[IBIS VER]   5.0
[File Name]   am13e230pzh.ibs
[File Rev]   1.0
[Date]   February 08, 2026
[Source]   File originated at Texas Instruments
[Copyright]   (c) 2012, Texas Instruments Inc.
[Component]   am13e230pzh
[Manufacturer] Texas Instruments
[Package]
| Variable   Typ   Min   Max
   R_pkg 3.31E-01 5.89E-02 4.13E-01
   L_pkg 7.43E-09 3.45E-09 1.00E-08
   C_pkg 1.76E-14 8.71E-15 4.53E-14
[Pin]   signal_name   model_name   R_pin   L_pin   C_pin
   1   PC2   BCF3385DSHYPBFZSD_87U 3.83E-01 8.46E-09 3.97E-14
   2   PC3   BCF3385DSHYPBFZSD_87U 3.62E-01 8.13E-09 1.93E-14
   3   PC4   BCF3385DSHYPBFZSD_87U 3.50E-01 7.91E-09 1.88E-14
   4   PC5   BCF3385DSHYPBFZSD_87U 3.41E-01 7.70E-09 1.83E-14
   5   PC6   BCF3385DSWHYPBFZSD_87U 3.34E-01 7.52E-09 1.78E-14
   6   VDD   NC 3.34E-01 7.42E-09 1.74E-14
   7   PB13   BCF3385DSWHYPBFZSD_87U 3.26E-01 7.22E-09 1.70E-14
   8   PB14   BCF3385DSHYPBFZSD_87U 3.24E-01 7.10E-09 1.66E-14
   9   PB15   BCF3385DSHYPBFZSD_87U 3.23E-01 6.98E-09 1.61E-14
   10   VSS   NC 3.28E-01 6.93E-09 1.58E-14
   11   VDD   NC 3.30E-01 6.83E-09 1.54E-14
   12 PC16_X1   BCF3385DSHYPBFZSD_87U 3.24E-01 6.67E-09 1.81E-14
   13 PC17_X2   BCF3385DSHYPBFZSD_87U 3.22E-01 6.54E-09 1.76E-14
   14   NRST   BQ0491FSSD_XRSN_87U 3.25E-01 6.67E-09 1.81E-14
   15   PB0   BCF3385DSHYPBFZSD_87U 3.27E-01 6.80E-09 1.54E-14
   16   PB1   BCF3385DSWHYPBFZSD_87U 3.30E-01 6.94E-09 1.58E-14
   17   PB2   BCF3385DSHYPBFZSD_87U 3.34E-01 7.09E-09 1.62E-14
   18   PB3   BCF3385DSHYPBFZSD_87U 3.40E-01 7.26E-09 1.67E-14
   19   VSS   NC 3.52E-01 7.50E-09 1.72E-14
   20   VREFLO   NC 3.59E-01 7.67E-09 1.76E-14
   21   VREFHI   NC 3.56E-01 7.75E-09 1.80E-14
   22   VREFHI   NC 3.67E-01 7.97E-09 1.85E-14
   23   PA0   BCF3385DSWHYPBFZSD_87U 3.76E-01 8.17E-09 1.90E-14
   24   PA1   BCF3385DSHYPBFZSD_87U 3.89E-01 8.41E-09 1.95E-14
   25   PA2   BCF3385DSWHYPBFZSD_87U 4.05E-01 8.68E-09 4.00E-14
   26   PA3   BCF3385DSHYPBFZSD_87U 3.95E-01 1.00E-08 2.20E-14
   27   VSSA   NC 2.08E-01 7.97E-09 1.32E-14
   28   VDDA   NC 2.02E-01 7.77E-09 1.29E-14
   29   PA4   BCF3385DSHYPBFZSD_87U 3.48E-01 9.13E-09 1.01E-14
   30   PA5   BCF3385DSHYPBFZSD_87U 3.39E-01 8.90E-09 9.80E-15
   31   PA6   BCF3385DSHYPBFZSD_87U 3.33E-01 8.69E-09 9.56E-15
   32   PA7   BCF3385DSHYPBFZSD_87U 3.27E-01 8.49E-09 9.33E-15
   33   PB4   BCF3385DSHYPBFZSD_87U 3.24E-01 8.31E-09 9.11E-15
   34   PB5   BCF3385DSWHYPBFZSD_87U 3.22E-01 8.15E-09 8.90E-15
   35   PA16   BCF3385DSHYPBFZSD_87U 3.21E-01 8.00E-09 8.71E-15
   36   PA17   BCF3385DSHYPBFZSD_87U 3.22E-01 7.86E-09 1.95E-14
   37   PA18   BCF3385DSHYPBFZSD_87U 3.24E-01 7.74E-09 1.90E-14
   38   PC7   BCF3385DSHYPBFZSD_87U 3.27E-01 7.63E-09 1.85E-14
   39   PC8   BCF3385DSHYPBFZSD_87U 3.22E-01 7.44E-09 1.79E-14
   40   PC9   BCF3385DSHYPBFZSD_87U 3.18E-01 7.25E-09 1.73E-14
   41   PC10   BCF3385DSHYPBFZSD_87U 3.15E-01 7.08E-09 1.68E-14
   42   PC11   BCF3385DSHYPBFZSD_87U 3.14E-01 6.93E-09 1.62E-14
   43   PC12   BCF3385DSHYPBFZSD_87U 3.15E-01 6.80E-09 1.57E-14
   44   PC13   BCF3385DSHYPBFZSD_87U 3.17E-01 6.68E-09 1.52E-14
   45   PC14   BCF3385DSHYPBFZSD_87U 3.21E-01 6.58E-09 1.78E-14
   46   PC15   BCF3385DSHYPBFZSD_87U 3.27E-01 6.49E-09 1.72E-14
   47   PA26   BCF3385DSHYPBFZSD_87U 3.34E-01 6.43E-09 1.66E-14
   48   NC   NC 5.89E-02 3.45E-09 1.38E-14
   49   VSS   NC 1.91E-01 4.66E-09 1.81E-14
   50   VDD   NC 3.69E-01 6.72E-09 2.96E-14
   51   PA28   BCF3385DSHYPBFZSD_87U 3.84E-01 8.47E-09 3.97E-14
   52   PA29   BCF3385DSHYPBFZSD_87U 3.71E-01 8.22E-09 1.93E-14
   53   PA30   BCF3385DSHYPBFZSD_87U 3.59E-01 8.00E-09 1.88E-14
   54   PA31   BCF3385DSHYPBFZSD_87U 3.49E-01 7.79E-09 1.84E-14
   55   PB24   BCF3385DSHYPBFZSD_87U 3.44E-01 7.62E-09 1.79E-14
   56   PB25   BCF3385DSHYPBFZSD_87U 3.37E-01 7.45E-09 1.75E-14
   57   PB26   BCF3385DSHYPBFZSD_87U 3.32E-01 7.29E-09 1.70E-14
   58   PB27   BCF3385DSHYPBFZSD_87U 3.28E-01 7.14E-09 1.66E-14
   59   PB28   BCF3385DSHYPBFZSD_87U 3.26E-01 7.01E-09 1.62E-14
   60   PB29   BCF3385DSHYPBFZSD_87U 3.24E-01 6.89E-09 1.58E-14
   61   PB30   BCF3385DSHYPBFZSD_87U 3.23E-01 6.77E-09 1.53E-14
   62   PB31   BCF3385DSHYPBFZSD_87U 3.24E-01 6.67E-09 1.81E-14
   63   PB6   BCF3385DSHYPBFZSD_87U 3.25E-01 6.57E-09 1.76E-14
   64   PB7   BCF3385DSHYPBFZSD_87U 3.27E-01 6.70E-09 1.81E-14
   65   PB8   BCF3385DSHYPBFZSD_87U 3.25E-01 6.79E-09 1.54E-14
   66   PB9   BCF3385DSHYPBFZSD_87U 3.28E-01 6.92E-09 1.58E-14
   67   PA8   BCF3385DSHYPBFZSD_87U 3.32E-01 7.07E-09 1.62E-14
   68   PA9   BCF3385DSHYPBFZSD_87U 3.37E-01 7.24E-09 1.67E-14
   69   PA10   BCF3385DSHYPBFZSD_87U 3.44E-01 7.41E-09 1.71E-14
   70   PA11   BCF3385DSHYPBFZSD_87U 3.40E-01 7.48E-09 1.75E-14
   71   PA12  BCPF335585DSHYPBFZSD_87U 3.48E-01 7.67E-09 1.80E-14
   72   PA13 BCF3385DSHYPBFZSD_TMS_87U 3.49E-01 7.78E-09 1.84E-14
   73   PC22   BCF3385DSHYPBFZSD_87U 3.59E-01 7.99E-09 1.88E-14
   74   VSS   NC 3.76E-01 8.28E-09 1.94E-14
   75   VDD   NC 2.10E-01 6.68E-09 4.53E-14
   76   PA14 BCF3385DSHYPBFZSD_TMS_87U 3.87E-01 9.96E-09 2.18E-14
   77   PA15  BCPF335585DSHYPBFZSD_87U 3.72E-01 9.67E-09 1.06E-14
   78   PB10   BCF3385DSHYPBFZSD_87U 3.60E-01 9.39E-09 1.03E-14
   79   PB11   BCF3385DSHYPBFZSD_87U 3.49E-01 9.14E-09 1.01E-14
   80   PB12   BCF3385DSHYPBFZSD_87U 3.40E-01 8.91E-09 9.80E-15
   81   PB16   BCF3385DSHYPBFZSD_87U 3.44E-01 8.80E-09 9.64E-15
   82   PB17   BCF3385DSHYPBFZSD_87U 3.36E-01 8.58E-09 9.39E-15
   83   PB18  BCPF335585DSHYPBFZSD_87U 3.35E-01 8.43E-09 9.20E-15
   84   PB19   BCF3385DSWHYPBFZSD_87U 3.31E-01 8.25E-09 8.98E-15
   85   PB20   BCF3385DSHYPBFZSD_87U 3.27E-01 8.06E-09 8.75E-15
   86   PB21   BCF3385DSHYPBFZSD_87U 3.23E-01 7.88E-09 1.95E-14
   87   PB22   BCF3385DSHYPBFZSD_87U 3.21E-01 7.72E-09 1.90E-14
   88   PB23   BCF3385DSHYPBFZSD_87U 3.21E-01 7.57E-09 1.84E-14
   89   PA19  BCPF335585DSHYPBFZSD_87U 3.20E-01 7.42E-09 1.79E-14
   90   PA20   BCF3385DSHYPBFZSD_87U 3.21E-01 7.28E-09 1.74E-14
   91   PA21   BCF3385DSHYPBFZSD_87U 3.20E-01 7.13E-09 1.68E-14
   92   PA22   BCF3385DSHYPBFZSD_87U 3.22E-01 7.01E-09 1.63E-14
   93   PA23   BCF3385DSHYPBFZSD_87U 3.26E-01 6.91E-09 1.58E-14
   94   PD11   BCF3385DSHYPBFZSD_87U 3.31E-01 6.82E-09 1.53E-14
   95   PA24   BCF3385DSHYPBFZSD_87U 3.38E-01 6.75E-09 1.79E-14
   96   PA25   BCF3385DSHYPBFZSD_87U 3.46E-01 6.69E-09 1.73E-14
   97   PC0   BCF3385DSHYPBFZSD_87U 3.56E-01 6.65E-09 1.67E-14
   98   PC1   BCF3385DSHYPBFZSD_87U 3.68E-01 6.64E-09 1.62E-14
   99   VSS   NC 2.01E-01 4.77E-09 1.84E-14
   100   VDD   NC 4.01E-01 7.05E-09 3.01E-14
| End of package information
|   Component BCF3385DSHYPBFZSD_87U
[Component] BCF3385DSHYPBFZSD_87U
[Manufacturer] Texas Instruments
[Package]
| variable   typ   min   max
R_pkg   0.0   0.0   0.0
L_pkg   0.0H   0.0H   0.0H
C_pkg   0.0F   0.0F   0.0F
[Pin]  signal_name   model_name   R_pin   L_pin   C_pin
PAD   PAD   BCF3385DSHYPBFZSD_87U
VDDS   VDDS   Power
VSS   VSS   Gnd
A   A   NC
GZ   GZ   NC
[Model Selector] BCF3385DSHYPBFZSD_87U
BCF3385DSHYPBFZSD_87U_PUPDOFF PI=1 PSEL=1
BCF3385DSHYPBFZSD_87U_PDON PI=0 PSEL=0
BCF3385DSHYPBFZSD_87U_PUON PI=0 PSEL=1
|   Component BCF3385DSHYPBFZSD_TMS_87U
[Component] BCF3385DSHYPBFZSD_TMS_87U
[Manufacturer] Texas Instruments
[Package]
| variable   typ   min   max
R_pkg   0.0   0.0   0.0
L_pkg   0.0H   0.0H   0.0H
C_pkg   0.0F   0.0F   0.0F
[Pin]  signal_name   model_name   R_pin   L_pin   C_pin
PAD   PAD   BCF3385DSHYPBFZSD_TMS_87U
VDDS   VDDS   Power
VSS   VSS   Gnd
A   A   NC
GZ   GZ   NC
[Model Selector] BCF3385DSHYPBFZSD_TMS_87U
BCF3385DSHYPBFZSD_TMS_87U_PUPDOFF PI=1 PSEL=1
BCF3385DSHYPBFZSD_TMS_87U_PDON PI=0 PSEL=0
BCF3385DSHYPBFZSD_TMS_87U_PUON PI=0 PSEL=1
|   Component BCF3385DSWHYPBFZSD_87U
[Component] BCF3385DSWHYPBFZSD_87U
[Manufacturer] Texas Instruments
[Package]
| variable   typ   min   max
R_pkg   0.0   0.0   0.0
L_pkg   0.0H   0.0H   0.0H
C_pkg   0.0F   0.0F   0.0F
[Pin]  signal_name   model_name   R_pin   L_pin   C_pin
PAD   PAD   BCF3385DSWHYPBFZSD_87U
VDDS   VDDS   Power
VSS   VSS   Gnd
A   A   NC
GZ   GZ   NC
[Model Selector] BCF3385DSWHYPBFZSD_87U
BCF3385DSWHYPBFZSD_87U_PUPDOFF PI=1 PSEL=1
BCF3385DSWHYPBFZSD_87U_PDON PI=0 PSEL=0
BCF3385DSWHYPBFZSD_87U_PUON PI=0 PSEL=1
|   Component BCPF335585DSHYPBFZSD_87U
[Component] BCPF335585DSHYPBFZSD_87U
[Manufacturer] Texas Instruments
[Package]
| variable   typ   min   max
R_pkg   0.0   0.0   0.0
L_pkg   0.0H   0.0H   0.0H
C_pkg   0.0F   0.0F   0.0F
[Pin]  signal_name   model_name   R_pin   L_pin   C_pin
PAD   PAD   BCPF335585DSHYPBFZSD_87U
VDDS   VDDS   Power
VSS   VSS   Gnd
A   A   NC
GZ   GZ   NC
[Model Selector] BCPF335585DSHYPBFZSD_87U
BCPF335585DSHYPBFZSD_87U_PUPDOFF_D0 DS=0
BCPF335585DSHYPBFZSD_87U_PUPDOFF_D1 DS=1
BCPF335585DSHYPBFZSD_87U_PDON PI=0 PSEL=0
BCPF335585DSHYPBFZSD_87U_PUON PI=0 PSEL=1
|   Component BQ0491FSSD_XRSN_87U
[Component] BQ0491FSSD_XRSN_87U
[Manufacturer] Texas Instruments
[Package]
| variable   typ   min   max
R_pkg   0.0   0.0   0.0
L_pkg   0.0H   0.0H   0.0H
C_pkg   0.0F   0.0F   0.0F
[Pin]  signal_name   model_name   R_pin   L_pin   C_pin
PAD   PAD   BQ0491FSSD_XRSN_87U
VDDS   VDDS   Power
VSS   VSS   Gnd
A   A   NC
[Model Selector] BQ0491FSSD_XRSN_87U
BQ0491FSSD_XRSN_87U_PUPDOFF PI=1
BQ0491FSSD_XRSN_87U_PUPDON PI=0
| Models and submodels in the file (15): BCF3385DSHYPBFZSD_87U_PUPDOFF (I/O), BCF3385DSHYPBFZSD_87U_PDON (Input), BCF3385DSHYPBFZSD_87U_PUON (Input), BCF3385DSHYPBFZSD_TMS_87U_PUPDOFF (I/O), BCF3385DSHYPBFZSD_TMS_87U_PDON (Input), BCF3385DSHYPBFZSD_TMS_87U_PUON (Input), BCF3385DSWHYPBFZSD_87U_PUPDOFF (I/O), BCF3385DSWHYPBFZSD_87U_PDON (Input), BCF3385DSWHYPBFZSD_87U_PUON (Input), BCPF335585DSHYPBFZSD_87U_PUPDOFF_D0 (I/O), BCPF335585DSHYPBFZSD_87U_PUPDOFF_D1 (I/O), BCPF335585DSHYPBFZSD_87U_PDON (Input), BCPF335585DSHYPBFZSD_87U_PUON (Input), BQ0491FSSD_XRSN_87U_PUPDOFF (Input), BQ0491FSSD_XRSN_87U_PUPDON (Input)
